| IBIS file generated by  Version 3.24
|   j6plus
[IBIS ver]   5.0
[File name]   j6plus.ibs
[File Rev]   1.0.0
[Date]   Mon Apr 10, 2017, 14:43:27
[Source]   Data created at Texas Instruments
[Notes]   J6Plus 23mm IBIS Model Revision History
   Version 1.0.0, April 10th, 2017
   - Initial Release
   Note 1) Checked by IBISCHK5.
[Disclaimer] Please be aware that in the absence of a written agreement,
   Texas Instruments (TI) assumes no liability for: 1) the
   accuracy of the IBIS models provided to your company, 2) the
   proper functioning of these IBIS models in your design or for
   any resulting applications, or, 3) infringement of patents,
   copyrights, or intellectual property rights resulting from
   your use of these IBIS models. TI provides IBIS models as a
   service to our customers and therefore reserves the right to
   limit distribution of the IBIS models.
[Copyright]   Property of Texas Instruments Incorporated. Unauthorised
   reproduction and/or distribution is strictly prohibited. This
   product is protected under copyright law and trade secret law
   as an unpublished work. Created 2016,(C) Copyright 2016,
   Texas Instruments Incorporated., All Rights Reserved. These
   commodities are under the U.S. Government distribution license
   control.As such,they are not to be re-exported without the
   prior approval of the U.S. Department of Commerce.
|   Component j6plus
[Component]   j6plus
[Manufacturer]   Texas Instruments.
| Source IO level model revisions
|Model   Revision   Date
|DDR_SEIOPB_H   2.5   23 May 2014
|CAMERARX_ADDON   0.9   March 31, 2014
|ACSPCIE_RX   0.5   May 16, 2012
|HDMITXPHY   0.8   Jul 12, 2011
|BC1833DV40DCPBFBP1811_SSCEH   2.0   Sep 11, 2013
|CAMERARX_CORE   0.9   March 31, 2014
|IQ1833DVTCKPBFBP18LL_SSCEV   2.0   Sep 11, 2013
|SDIO1833PB_H   1.0   Sep 21, 2011
|DDR_SEIOPB_V   2.5   23 May 2014
|IHHV1833DVHYP1811_SSCEV   1.0   Dec 24, 2012
|DDR_DIFFIOPB_V   2.5   23 May 2014
|BI2C1833DVFZP18_SSCEV   2.0   Sep 11, 2013
|GANGARX   1   Sep 04, 2012
|SATATX   1.0   Nov 07, 2012
|USB3_PCIEGEN1_PCIEGEN2_TX   1.0   Nov 07, 2012
|DDR_DIFFIOPB_H   2.5   23 May 2014
|BC1833DV40DCPBFBP1811_SSCEV   2.0   Sep 11, 2013
|USB2PHYCORE_HMAV10GS80   0.8   July 13, 2011
|BMLBLVDS18_SSCEH   1.0   Jun 13, 2013
[Package]
|   typ   min   max
R_pkg   0.42369669665272   0.092871   0.97124
L_pkg   2.90117154811716E-009 1.36E-09   4.86E-09
C_pkg   1.52619874476987E-012 8.24E-13   2.21E-12
[Pin]   signal_name   model_name   R_pin   L_pin   C_pin
F6   ATESTV   NC
AC17   CSI2_1_DY2   Selector_15  0.47322   3.10E-09   1.23E-12
AE16   CSI2_0_DY3   Selector_17  0.44019   2.71E-09   1.13E-12
AC13   CSI2_1_DX0   Selector_25  0.46457   2.78E-09   1.07E-12
AF16   CSI2_0_DX1   Selector_13  0.50237   2.99E-09   1.30E-12
AD15   CSI2_1_DX1   Selector_13  0.40521   2.59E-09   1.12E-12
AD17   CSI2_0_DX0   Selector_25  0.3281   2.01E-09   9.66E-13
AF19   CSI2_0_DX2   Selector_13  0.5902   3.45E-09   1.35E-12
AE18   CSI2_0_DY4   Selector_17  0.49636   2.64E-09   1.25E-12
AF17   CSI2_0_DY1   Selector_15  0.50908   3.01E-09   1.32E-12
AD14   CSI2_1_DY1   Selector_15  0.4246   2.63E-09   1.07E-12
AD18   CSI2_0_DY0   Selector_17  0.31895   1.98E-09   9.93E-13
AC16   CSI2_1_DX2   Selector_13  0.47087   3.11E-09   1.25E-12
AE19   CSI2_0_DX4   Selector_25  0.4925   2.76E-09   1.18E-12
AE15   CSI2_0_DX3   Selector_25  0.43712   2.72E-09   1.11E-12
AC14   CSI2_1_DY0   Selector_17  0.46446   2.94E-09   1.04E-12
AF20   CSI2_0_DY2   Selector_15  0.60517   3.60E-09   1.40E-12
E19   DCAN1_TX   Selector_23  0.17732   1.75E-09   1.07E-12
D19   DCAN1_RX   Selector_23  0.29009   2.59E-09   1.21E-12
AA27   DDR1_D20   Selector_24  0.47426   3.29E-09   1.74E-12
AB22   DDR1_VREF0   NC
AA24   DDR1_D21   Selector_24  0.33247   2.23E-09   1.42E-12
AH23   DDR1_CKE   Selector_22  0.54196   3.53E-09   1.79E-12
AC28   DDR1_DQSN1   Selector_26  0.65798   3.81E-09   1.48E-12
V28   DDR1_ECC_D7   Selector_24  0.47152   3.15E-09   1.68E-12
AE24   DDR1_A11   Selector_22  0.35245   2.44E-09   1.42E-12
W25   DDR1_D28   Selector_24  0.28879   2.13E-09   1.29E-12
AF22   DDR1_ODT0   Selector_22  0.40147   2.81E-09   1.44E-12
AB27   DDR1_DQS2   Selector_20  0.67189   3.76E-09   1.46E-12
AE25   DDR1_D13   Selector_24  0.41515   3.01E-09   1.57E-12
Y24   DDR1_D27   Selector_24  0.30467   2.05E-09   1.31E-12
AC27   DDR1_DQS1   Selector_20  0.67176   3.88E-09   1.45E-12
V25   DDR1_ECC_D2   Selector_24  0.35131   2.67E-09   1.44E-12
AF23   DDR1_RST   Selector_22  0.45466   3.02E-09   1.62E-12
AG23   DDR1_A8   Selector_22  0.42684   3.00E-09   1.61E-12
AB24   DDR1_D8   Selector_24  0.35689   2.67E-09   1.36E-12
AG26   DDR1_DQM0   Selector_11  0.64729   3.91E-09   2.00E-12
T27   DDR1_DQM_ECC   Selector_11  0.43684   3.03E-09   1.55E-12
AD28   DDR1_D11   Selector_24  0.53861   3.60E-09   1.82E-12
AE22   DDR1_A0   Selector_22  0.35492   2.49E-09   1.43E-12
AH25   DDR1_DQS0   Selector_20  0.68056   3.82E-09   1.46E-12
AC24   DDR1_DQM1   Selector_11  0.35873   2.52E-09   1.41E-12
AF21   DDR1_A13   Selector_22  0.38573   2.77E-09   1.62E-12
AG20   DDR1_A15   Selector_22  0.4557   3.04E-09   1.63E-12
AE20   DDR1_BA0   Selector_22  0.29234   2.04E-09   1.32E-12
AA28   DDR1_D19   Selector_24  0.49032   3.42E-09   1.85E-12
Y27   DDR1_DQM3   Selector_11  0.46763   3.07E-09   1.69E-12
AG21   DDR1_A12   Selector_22  0.38719   2.86E-09   1.64E-12
AG19   DDR1_CASN   Selector_22  0.42733   2.78E-09   1.62E-12
AD20   DDR1_A1   Selector_22  0.21926   1.63E-09   1.17E-12
AB25   DDR1_D17   Selector_24  0.40252   2.71E-09   1.56E-12
T28   DDR1_ECC_D5   Selector_24  0.44485   3.30E-09   1.71E-12
V26   DDR1_ECC_D3   Selector_24  0.33355   2.36E-09   1.48E-12
V24   DDR1_D26   Selector_24  0.26466   2.00E-09   1.29E-12
AF25   DDR1_D4   Selector_24  0.45643   3.11E-09   1.58E-12
AB26   DDR1_DQM2   Selector_11  0.41898   2.75E-09   1.59E-12
AD24   DDR1_A6   Selector_22  0.35013   2.68E-09   1.63E-12
AG22   DDR1_WEN   Selector_22  0.42447   2.86E-09   1.58E-12
AE27   DDR1_D1   Selector_24  0.52049   3.42E-09   1.76E-12
AC26   DDR1_D15   Selector_24  0.41191   2.78E-09   1.58E-12
T26   DDR1_ECC_D6   Selector_24  0.34602   2.50E-09   1.43E-12
AD25   DDR1_D14   Selector_24  0.39609   2.83E-09   1.50E-12
AE21   DDR1_A2   Selector_22  0.28785   2.13E-09   1.21E-12
AC22   DDR1_A7   Selector_22  0.22439   1.72E-09   1.21E-12
AF26   DDR1_D7   Selector_24  0.45878   3.16E-09   1.64E-12
AF28   DDR1_D2   Selector_24  0.62581   3.95E-09   1.94E-12
AB23   DDR1_D25   Selector_24  0.34495   2.49E-09   1.54E-12
U26   DDR1_ECC_D1   Selector_24  0.34279   2.39E-09   1.49E-12
AH24   DDR1_NCK   Selector_1   0.6371   3.54E-09   1.68E-12
U27   DDR1_DQS_ECC   Selector_20  0.5902   3.35E-09   1.36E-12
AE26   DDR1_D0   Selector_24  0.50411   3.40E-09   1.67E-12
AD23   DDR1_CSN0   Selector_22  0.31244   2.34E-09   1.50E-12
AD22   DDR1_A3   Selector_22  0.27077   2.08E-09   1.24E-12
W24   DDR1_D30   Selector_24  0.3292   2.27E-09   1.37E-12
AC25   DDR1_D22   Selector_24  0.46439   3.12E-09   1.76E-12
AH22   DDR1_A5   Selector_22  0.48585   3.28E-09   1.74E-12
AG24   DDR1_CK   Selector_6   0.63186   3.52E-09   1.69E-12
AB28   DDR1_DQSN2   Selector_26  0.66433   3.80E-09   1.48E-12
AD26   DDR1_D12   Selector_24  0.44133   3.15E-09   1.59E-12
AF27   DDR1_D6   Selector_24  0.53391   3.62E-09   1.76E-12
V27   DDR1_ECC_D4   Selector_24  0.41597   2.89E-09   1.57E-12
AE23   DDR1_A4   Selector_22  0.37808   2.74E-09   1.49E-12
U25   DDR1_ECC_D0   Selector_24  0.30068   2.13E-09   1.30E-12
AF24   DDR1_A9   Selector_22  0.39658   2.69E-09   1.50E-12
AH26   DDR1_D3   Selector_24  0.58696   3.71E-09   1.90E-12
AE28   DDR1_D10   Selector_24  0.59778   3.95E-09   1.91E-12
W26   DDR1_D24   Selector_24  0.41375   2.90E-09   1.50E-12
Y28   DDR1_D31   Selector_24  0.48908   3.29E-09   1.77E-12
AD21   DDR1_A10   Selector_22  0.18857   1.54E-09   1.06E-12
AH20   DDR1_RASN   Selector_22  0.45523   2.97E-09   1.68E-12
AG27   DDR1_D5   Selector_24  0.5732   3.45E-09   1.89E-12
AA25   DDR1_D16   Selector_24  0.40361   2.85E-09   1.49E-12
AC23   DDR1_A14   Selector_22  0.36157   2.89E-09   1.65E-12
AH21   DDR1_BA2   Selector_22  0.50674   3.32E-09   1.77E-12
Y26   DDR1_D23   Selector_24  0.30563   2.40E-09   1.43E-12
AG25   DDR1_DQSN0   Selector_26  0.66118   3.82E-09   1.45E-12
Y25   DDR1_D29   Selector_24  0.33786   2.36E-09   1.34E-12
AA26   DDR1_D18   Selector_24  0.40984   2.78E-09   1.59E-12
U28   DDR1_DQSN_ECC   Selector_26  0.58142   3.43E-09   1.36E-12
AD27   DDR1_D9   Selector_24  0.46233   3.31E-09   1.75E-12
W27   DDR1_DQSN3   Selector_26  0.62804   3.57E-09   1.42E-12
W28   DDR1_DQS3   Selector_20  0.65151   3.67E-09   1.43E-12
AC21   DDR1_BA1   Selector_22  0.20841   1.95E-09   1.21E-12
P23   DDR2_A5   Selector_11  0.19884   1.81E-09   1.27E-12
M24   DDR2_BA2   Selector_11  0.38561   3.08E-09   1.66E-12
H25   DDR2_D21   Selector_24  0.32873   2.40E-09   1.46E-12
B27   DDR2_D5   Selector_24  0.52339   3.75E-09   2.03E-12
H27   DDR2_D22   Selector_24  0.44149   3.11E-09   1.66E-12
N24   DDR2_A14   Selector_11  0.20496   1.86E-09   1.20E-12
T25   DDR2_CASN   Selector_11  0.2726   2.24E-09   1.19E-12
R24   DDR2_A13   Selector_11  0.19051   1.48E-09   1.02E-12
R25   DDR2_CKE   Selector_11  0.32341   2.57E-09   1.33E-12
J28   DDR2_DQSN2   Selector_26  0.59604   3.55E-09   1.37E-12
E25   DDR2_D9   Selector_24  0.36266   2.71E-09   1.47E-12
R28   DDR2_CK   Selector_14  0.63061   3.59E-09   1.61E-12
K24   DDR2_D30   Selector_24  0.22548   2.13E-09   1.35E-12
G27   DDR2_D11   Selector_24  0.43022   3.03E-09   1.58E-12
K26   DDR2_D25   Selector_24  0.36091   2.55E-09   1.44E-12
L28   DDR2_DQS3   Selector_20  0.62529   3.80E-09   1.40E-12
J24   DDR2_D29   Selector_24  0.27245   2.16E-09   1.35E-12
N25   DDR2_RST   Selector_11  0.33044   2.79E-09   1.43E-12
J25   DDR2_D26   Selector_24  0.35274   2.47E-09   1.39E-12
T24   DDR2_WEN   Selector_11  0.23939   1.92E-09   1.18E-12
J27   DDR2_DQS2   Selector_20  0.604   3.52E-09   1.34E-12
P26   DDR2_A1   Selector_11  0.35121   2.52E-09   1.45E-12
H24   DDR2_D28   Selector_24  0.33905   2.66E-09   1.59E-12
N26   DDR2_A6   Selector_11  0.3636   2.64E-09   1.45E-12
F27   DDR2_DQS1   Selector_20  0.7305   4.09E-09   1.57E-12
L25   DDR2_A10   Selector_11  0.3358   2.53E-09   1.53E-12
D26   DDR2_D4   Selector_24  0.44637   3.26E-09   1.60E-12
R26   DDR2_RASN   Selector_11  0.32251   2.49E-09   1.34E-12
K28   DDR2_D27   Selector_24  0.47179   3.20E-09   1.69E-12
R23   DDR2_A15   Selector_11  0.17102   1.42E-09   9.48E-13
M27   DDR2_A9   Selector_11  0.4387   3.07E-09   1.64E-12
D25   DDR2_D3   Selector_24  0.39925   2.89E-09   1.49E-12
K27   DDR2_D24   Selector_24  0.45334   3.19E-09   1.58E-12
D27   DDR2_DQSN0   Selector_26  0.68594   3.95E-09   1.46E-12
P28   DDR2_A2   Selector_11  0.4806   3.52E-09   1.80E-12
J26   DDR2_DQM3   Selector_11  0.42358   3.15E-09   1.66E-12
H28   DDR2_D20   Selector_24  0.49628   3.66E-09   1.84E-12
P27   DDR2_A3   Selector_11  0.40859   2.90E-09   1.58E-12
G24   DDR2_D17   Selector_24  0.35079   2.66E-09   1.60E-12
P25   DDR2_A0   Selector_11  0.26462   2.02E-09   1.23E-12
A26   DDR2_D1   Selector_24  0.50901   3.87E-09   2.00E-12
E24   DDR2_D2   Selector_24  0.38689   2.96E-09   1.52E-12
U24   DDR2_BA1   Selector_11  0.26815   2.12E-09   1.21E-12
C26   DDR2_D7   Selector_24  0.45744   3.30E-09   1.76E-12
M22   DDR2_VREF0   NC
M25   DDR2_A7   Selector_11  0.26291   2.06E-09   1.30E-12
F24   DDR2_D19   Selector_24  0.34822   2.79E-09   1.70E-12
G23   DDR2_DQM2   Selector_11  0.27859   2.26E-09   1.57E-12
C28   DDR2_D0   Selector_24  0.62669   4.38E-09   2.04E-12
M26   DDR2_CSN0   Selector_11  0.33733   2.53E-09   1.55E-12
F26   DDR2_D8   Selector_24  0.43184   3.11E-09   1.46E-12
P24   DDR2_A4   Selector_11  0.20852   1.74E-09   1.08E-12
E26   DDR2_D10   Selector_24  0.45673   3.22E-09   1.56E-12
F23   DDR2_D18   Selector_24  0.32703   2.83E-09   1.75E-12
B26   DDR2_D6   Selector_24  0.50709   3.63E-09   1.97E-12
E28   DDR2_D12   Selector_24  0.57819   3.92E-09   1.81E-12
D28   DDR2_DQS0   Selector_20  0.71828   4.02E-09   1.50E-12
N28   DDR2_A8   Selector_11  0.48119   3.33E-09   1.70E-12
K25   DDR2_ODT0   Selector_11  0.445   3.37E-09   1.86E-12
L27   DDR2_DQSN3   Selector_26  0.60186   3.60E-09   1.43E-12
G25   DDR2_D16   Selector_24  0.41288   3.08E-09   1.71E-12
F28   DDR2_DQSN1   Selector_26  0.73785   4.21E-09   1.57E-12
G28   DDR2_D14   Selector_24  0.4674   3.37E-09   1.76E-12
L26   DDR2_D31   Selector_24  0.34691   2.45E-09   1.41E-12
N27   DDR2_A11   Selector_11  0.38845   2.75E-09   1.51E-12
H26   DDR2_D23   Selector_24  0.37415   2.64E-09   1.56E-12
F25   DDR2_D15   Selector_24  0.34955   2.65E-09   1.39E-12
C27   DDR2_DQM0   Selector_11  0.5469   4.01E-09   1.82E-12
L24   DDR2_BA0   Selector_11  0.2659   2.36E-09   1.44E-12
G26   DDR2_D13   Selector_24  0.38989   2.74E-09   1.55E-12
E27   DDR2_DQM1   Selector_11  0.55797   3.78E-09   1.97E-12
M28   DDR2_A12   Selector_11  0.47329   3.27E-09   1.73E-12
R27   DDR2_NCK   Selector_27  0.61545   3.53E-09   1.63E-12
F19   EMU0   Selector_23  0.13176   1.42E-09   8.78E-13
C23   EMU1   Selector_23  0.51333   3.38E-09   1.80E-12
F17   GPIO6_15   Selector_23  0.19784   1.98E-09   1.08E-12
AB4   GPIO6_11   Selector_4   0.46323   2.99E-09   1.77E-12
AC5   GPIO6_10   Selector_4   0.61618   3.82E-09   2.06E-12
F18   GPIO6_16   Selector_23  0.15426   1.52E-09   9.50E-13
E21   GPIO6_14   Selector_23  0.25374   2.28E-09   1.07E-12
R1   GPMC_A18   Selector_4   0.49354   3.50E-09   1.72E-12
M5   GPMC_OEN_REN   Selector_4   0.25199   2.05E-09   1.12E-12
H5   GPMC_A27   Selector_4   0.22331   1.86E-09   1.13E-12
P6   GPMC_A0   Selector_4   0.18008   1.52E-09   1.09E-12
L5   GPMC_AD2   Selector_4   0.26493   2.15E-09   1.15E-12
M4   GPMC_BEN1   Selector_4   0.28629   2.30E-09   1.24E-12
K2   GPMC_AD13   Selector_4   0.36396   2.68E-09   1.47E-12
T2   GPMC_A15   Selector_4   0.53356   3.66E-09   1.78E-12
L1   GPMC_AD8   Selector_4   0.50617   3.58E-09   1.67E-12
H4   GPMC_A25   Selector_4   0.28037   2.27E-09   1.33E-12
J2   GPMC_AD11   Selector_4   0.42103   3.01E-09   1.57E-12
K6   GPMC_AD4   Selector_4   0.23005   1.89E-09   1.10E-12
M2   GPMC_AD1   Selector_4   0.41338   3.06E-09   1.55E-12
J1   GPMC_AD10   Selector_4   0.498   3.50E-09   1.70E-12
P3   GPMC_A17   Selector_4   0.41172   2.97E-09   1.54E-12
G4   GPMC_CS1   Selector_4   0.26966   2.20E-09   1.26E-12
M1   GPMC_AD3   Selector_4   0.48001   3.52E-09   1.67E-12
G5   GPMC_A23   Selector_4   0.22275   2.08E-09   1.21E-12
R4   GPMC_A2   Selector_4   0.34771   2.60E-09   1.14E-12
J5   GPMC_A10   Selector_4   0.22191   2.40E-09   1.28E-12
M3   GPMC_WEN   Selector_4   0.34292   2.82E-09   1.36E-12
H1   GPMC_AD12   Selector_4   0.5391   3.75E-09   1.75E-12
N4   GPMC_A8   Selector_4   0.27934   2.32E-09   1.23E-12
L4   GPMC_AD5   Selector_4   0.25799   2.02E-09   1.23E-12
N2   GPMC_WAIT0   Selector_4   0.41982   3.14E-09   1.53E-12
N5   GPMC_AD0   Selector_4   0.40226   3.08E-09   1.52E-12
J6   GPMC_A1   Selector_4   0.23468   2.46E-09   1.24E-12
H6   GPMC_A19   Selector_4   0.15553   1.39E-09   8.82E-13
H2   GPMC_AD14   Selector_4   0.49023   3.33E-09   1.65E-12
P2   GPMC_CS2   Selector_4   0.43903   3.14E-09   1.57E-12
U1   GPMC_A16   Selector_4   0.54425   3.76E-09   1.82E-12
H3   GPMC_A26   Selector_4   0.31252   2.45E-09   1.40E-12
J3   GPMC_A24   Selector_4   0.31402   2.52E-09   1.35E-12
F5   GPMC_A22   Selector_4   0.28715   2.79E-09   1.47E-12
K5   GPMC_A11   Selector_4   0.23539   2.44E-09   1.27E-12
N6   GPMC_A7   Selector_4   0.17847   1.50E-09   1.02E-12
R2   GPMC_A13   Selector_4   0.43208   3.16E-09   1.59E-12
L2   GPMC_AD7   Selector_4   0.40505   2.94E-09   1.55E-12
K3   GPMC_AD15   Selector_4   0.30569   2.36E-09   1.34E-12
G6   GPMC_A20   Selector_4   0.22002   1.98E-09   1.24E-12
R3   GPMC_A9   Selector_4   0.40041   2.92E-09   1.50E-12
K4   GPMC_A5   Selector_4   0.31091   2.86E-09   1.40E-12
J4   GPMC_A21   Selector_4   0.24739   2.01E-09   1.27E-12
L3   GPMC_AD6   Selector_4   0.38163   2.77E-09   1.43E-12
N3   GPMC_BEN0   Selector_4   0.29182   2.53E-09   1.32E-12
K1   GPMC_AD9   Selector_4   0.40967   2.97E-09   1.58E-12
R5   GPMC_A3   Selector_4   0.26198   2.01E-09   1.09E-12
P1   GPMC_CS3   Selector_4   0.54568   3.87E-09   1.77E-12
P5   GPMC_A6   Selector_4   0.34047   2.61E-09   1.32E-12
R6   GPMC_A14   Selector_4   0.44443   3.33E-09   1.69E-12
P4   GPMC_A12   Selector_4   0.29397   2.27E-09   1.32E-12
L6   GPMC_CLK   Selector_4   0.16087   1.50E-09   1.26E-12
M6   GPMC_A4   Selector_4   0.15466   1.38E-09   1.02E-12
N1   GPMC_ADVN_ALE   Selector_4   0.52762   3.88E-09   1.73E-12
T1   GPMC_CS0   Selector_4   0.5994   4.10E-09   1.89E-12
AG14   HDMI1_CLOCKX   ibis_tmdsp_M#336   0.55573   2.99E-09   1.37E-12
AH18   HDMI1_DATA1Y   ibis_tmdsm_M#337   0.59298   3.19E-09   1.39E-12
AG18   HDMI1_DATA2X   ibis_tmdsp_M#336   0.56768   3.10E-09   1.28E-12
AH16   HDMI1_DATA0Y   ibis_tmdsm_M#337   0.52675   2.88E-09   1.32E-12
AG15   HDMI1_DATA0X   ibis_tmdsp_M#336   0.52784   2.86E-09   1.33E-12
AG17   HDMI1_DATA1X   ibis_tmdsp_M#336   0.56542   3.06E-09   1.37E-12
AH19   HDMI1_DATA2Y   ibis_tmdsm_M#337   0.58397   3.26E-09   1.31E-12
AH15   HDMI1_CLOCKY   ibis_tmdsm_M#337   0.55862   3.05E-09   1.37E-12
C19   I2C1_SCL   Selector_16  0.37854   2.73E-09   1.57E-12
C20   I2C1_SDA   Selector_16  0.41108   2.82E-09   1.55E-12
F15   I2C2_SCL   Selector_16  0.24519   2.03E-09   1.36E-12
C24   I2C2_SDA   Selector_16  0.56681   3.51E-09   1.90E-12
B28   IFORCE   NC
AF14   LJCB_CLKN   ACSPCIE_RX_M#335   0.3515   1.98E-09   1.29E-12
AE13   LJCB_CLKP   ACSPCIE_RX_M#335   0.35246   1.95E-09   1.29E-12
C12   MCASP1_AXR10   Selector_23  0.33446   2.49E-09   1.47E-12
D14   MCASP1_AXR12   Selector_23  0.22318   1.95E-09   1.22E-12
E12   MCASP1_AXR4   Selector_23  0.21323   1.78E-09   1.17E-12
D13   MCASP1_AXR5   Selector_23  0.23567   2.08E-09   1.21E-12
B12   MCASP1_AXR13   Selector_23  0.42421   3.04E-09   1.58E-12
B11   MCASP1_AXR8   Selector_23  0.38326   2.96E-09   1.57E-12
E14   MCASP1_AXR15   Selector_23  0.24085   1.99E-09   1.16E-12
A12   MCASP1_AXR11   Selector_23  0.45509   3.30E-09   1.65E-12
A11   MCASP1_AXR9   Selector_23  0.46183   3.35E-09   1.68E-12
E11   MCASP1_AXR3   Selector_23  0.25365   2.05E-09   1.24E-12
D12   MCASP1_AXR7   Selector_23  0.30704   2.35E-09   1.28E-12
B13   MCASP1_ACLKX   Selector_23  0.38146   2.87E-09   1.53E-12
C11   MCASP1_AXR6   Selector_23  0.32814   2.57E-09   1.43E-12
F11   MCASP1_AXR1   Selector_23  0.21935   1.87E-09   1.14E-12
C13   MCASP1_FSX   Selector_23  0.26929   2.19E-09   1.39E-12
F14   MCASP1_FSR   Selector_23  0.18526   1.56E-09   1.07E-12
A13   MCASP1_ACLKR   Selector_23  0.42105   3.00E-09   1.63E-12
E13   MCASP1_AXR2   Selector_23  0.092871   1.38E-09   8.93E-13
F12   MCASP1_AXR14   Selector_23  0.17677   1.62E-09   8.24E-13
F10   MCASP1_AXR0   Selector_23  0.18905   1.82E-09   1.19E-12
A17   MCASP2_FSX   Selector_23  0.58524   3.96E-09   2.02E-12
A19   MCASP2_FSR   Selector_23  0.65208   4.23E-09   2.18E-12
A16   MCASP2_AXR7   Selector_23  0.552   3.72E-09   1.93E-12
B14   MCASP2_AXR0   Selector_23  0.39699   2.82E-09   1.66E-12
B15   MCASP2_AXR5   Selector_23  0.44426   3.16E-09   1.66E-12
A14   MCASP2_AXR1   Selector_23  0.50121   3.46E-09   1.75E-12
D15   MCASP2_AXR4   Selector_23  0.28214   2.20E-09   1.35E-12
A15   MCASP2_AXR3   Selector_23  0.48973   3.34E-09   1.74E-12
C14   MCASP2_AXR2   Selector_23  0.32212   2.37E-09   1.39E-12
A18   MCASP2_ACLKX   Selector_23  0.53013   3.51E-09   1.84E-12
B16   MCASP2_AXR6   Selector_23  0.39   2.84E-09   1.58E-12
E15   MCASP2_ACLKR   Selector_23  0.1899   1.46E-09   1.15E-12
B18   MCASP3_AXR0   Selector_23  0.41165   2.85E-09   1.57E-12
B17   MCASP3_ACLKX   Selector_23  0.42894   2.91E-09   1.63E-12
C16   MCASP3_AXR1   Selector_23  0.34144   2.49E-09   1.45E-12
F13   MCASP3_FSX   Selector_23  0.23996   2.05E-09   1.21E-12
A20   MCASP4_FSX   Selector_23  0.52153   3.48E-09   1.82E-12
D17   MCASP4_AXR1   Selector_23  0.27464   2.06E-09   1.30E-12
D16   MCASP4_AXR0   Selector_23  0.16794   1.84E-09   1.18E-12
C17   MCASP4_ACLKX   Selector_23  0.4215   2.91E-09   1.52E-12
AB6   MCASP5_FSX   Selector_4   0.41465   2.73E-09   1.58E-12
AA4   MCASP5_AXR1   Selector_4   0.43954   2.86E-09   1.74E-12
AB3   MCASP5_AXR0   Selector_4   0.46779   3.05E-09   1.77E-12
AA3   MCASP5_ACLKX   Selector_4   0.4844   3.22E-09   1.67E-12
V1   MDIO_MCLK   Selector_4   0.57447   3.80E-09   1.90E-12
U3   MDIO_D   Selector_4   0.38305   2.58E-09   1.53E-12
AB1   MLBP_CLK_P   Selector_2   0.7668   4.20E-09   1.85E-12
AA2   MLBP_DAT_N   Selector_9   0.72941   4.04E-09   1.52E-12
AB2   MLBP_CLK_N   Selector_2   0.76043   4.14E-09   1.83E-12
AC2   MLBP_SIG_N   Selector_9   0.78823   4.31E-09   1.59E-12
AA1   MLBP_DAT_P   Selector_9   0.72772   4.13E-09   1.51E-12
AC1   MLBP_SIG_P   Selector_9   0.80114   4.31E-09   1.63E-12
V6   MMC1_SDWP   Selector_4   0.19952   1.46E-09   1.16E-12
W3   MMC1_CLK   Selector_5   0.36035   2.56E-09   1.58E-12
W4   MMC1_SDCD   Selector_4   0.31882   2.24E-09   1.44E-12
Y4   MMC1_DAT1   Selector_5   0.40029   2.71E-09   1.67E-12
V5   MMC1_DAT0   Selector_5   0.31001   2.32E-09   1.34E-12
Y3   MMC1_DAT3   Selector_5   0.42805   2.91E-09   1.61E-12
W5   MMC1_CMD   Selector_5   0.31704   2.16E-09   1.41E-12
Y5   MMC1_DAT2   Selector_5   0.39546   2.74E-09   1.64E-12
AB7   MMC3_DAT6   Selector_4   0.43055   2.92E-09   1.71E-12
AC6   MMC3_DAT2   Selector_4   0.46203   3.07E-09   1.66E-12
AC7   MMC3_CMD   Selector_4   0.5286   3.64E-09   1.84E-12
AC4   MMC3_DAT3   Selector_4   0.57319   3.45E-09   1.95E-12
AA5   MMC3_DAT7   Selector_4   0.35903   2.41E-09   1.52E-12
AA6   MMC3_DAT4   Selector_4   0.37993   2.63E-09   1.52E-12
AC3   MMC3_CLK   Selector_4   0.49296   3.15E-09   1.75E-12
AB5   MMC3_DAT5   Selector_4   0.38564   2.57E-09   1.54E-12
Y6   MMC3_DAT0   Selector_4   0.25419   1.80E-09   1.28E-12
W6   MMC3_DAT1   Selector_4   0.20733   1.58E-09   1.17E-12
AH9   PCIE_RXP1   usb3rx_M#715   0.65527   3.53E-09   1.47E-12
AG9   PCIE_TXN1   Selector_7   0.59952   3.27E-09   1.45E-12
AG12   PCIE_TXN0   Selector_7   0.52323   2.85E-09   1.33E-12
AH10   PCIE_TXP1   Selector_21  0.60849   3.34E-09   1.42E-12
AG11   PCIE_RXN0   usb3rx_M#715   0.52095   2.80E-09   1.33E-12
AG8   PCIE_RXN1   usb3rx_M#715   0.64833   3.44E-09   1.48E-12
AH12   PCIE_RXP0   usb3rx_M#715   0.52941   2.89E-09   1.33E-12
AH13   PCIE_TXP0   Selector_21  0.53798   2.89E-09   1.34E-12
C25   PORZ   Selector_18  0.53951   3.88E-09   1.78E-12
D24   RESETN   Selector_8   0.51082   3.80E-09   1.67E-12
T5   RGMII0_TXD0   Selector_4   0.2657   2.11E-09   1.25E-12
U4   RGMII0_RXC   Selector_4   0.40317   2.79E-09   1.56E-12
Y2   RGMII0_RXD1   Selector_4   0.59491   3.80E-09   1.90E-12
V4   RGMII0_RXCTL   Selector_4   0.40168   2.84E-09   1.60E-12
T4   RGMII0_TXD3   Selector_4   0.27961   2.19E-09   1.37E-12
W2   RGMII0_RXD3   Selector_4   0.5259   3.73E-09   1.81E-12
W1   RGMII0_RXD0   Selector_4   0.53313   3.74E-09   1.92E-12
T3   RGMII0_TXD2   Selector_4   0.34803   2.80E-09   1.51E-12
T6   RGMII0_TXC   Selector_4   0.18507   1.46E-09   1.13E-12
U5   RGMII0_TXCTL   Selector_4   0.33553   2.42E-09   1.33E-12
U6   RGMII0_TXD1   Selector_4   0.37411   2.67E-09   1.57E-12
V3   RGMII0_RXD2   Selector_4   0.44923   3.04E-09   1.70E-12
U2   RMII_MHZ_50_CLK   Selector_4   0.49781   3.29E-09   1.77E-12
D23   RSTOUTN   Selector_3   0.47264   3.40E-09   1.74E-12
E18   RTCK   Selector_3   0.20614   1.61E-09   1.14E-12
AG6   SATA1_TXN0   sata_tx_M#759   0.73959   3.93E-09   1.62E-12
AG5   SATA1_RXP0   usb3rx_M#715   0.83495   4.37E-09   1.75E-12
AH6   SATA1_RXN0   usb3rx_M#715   0.82304   4.33E-09   1.76E-12
AH7   SATA1_TXP0   sata_tx_M#759   0.7495   3.93E-09   1.61E-12
C15   SPI1_D1   Selector_23  0.17598   2.47E-09   1.35E-12
A21   SPI1_CS1   Selector_23  0.59228   3.79E-09   2.03E-12
B19   SPI1_CS3   Selector_23  0.47701   3.52E-09   1.86E-12
B24   SPI1_D0   Selector_23  0.34305   4.18E-09   2.17E-12
B20   SPI1_CS2   Selector_23  0.48542   3.52E-09   1.79E-12
A23   SPI1_CS0   Selector_23  0.62624   4.18E-09   2.08E-12
A24   SPI1_SCLK   Selector_23  0.70609   4.38E-09   2.17E-12
B23   SPI2_CS0   Selector_23  0.62835   3.92E-09   2.04E-12
E16   SPI2_D0   Selector_23  0.1358   1.46E-09   1.14E-12
B21   SPI2_D1   Selector_23  0.54119   3.70E-09   1.85E-12
A25   SPI2_SCLK   Selector_23  0.73945   4.49E-09   2.21E-12
E20   TCLK   Selector_12  0.23692   2.02E-09   1.14E-12
B22   TDI   Selector_8   0.44949   3.00E-09   1.76E-12
C18   TDO   Selector_3   0.27882   2.66E-09   1.29E-12
F16   TMS   Selector_23  0.20144   1.88E-09   1.16E-12
D20   TRSTN   Selector_8   0.30933   2.49E-09   1.30E-12
F22   UART1_RXD   Selector_23  0.24211   2.17E-09   1.16E-12
C21   UART1_TXD   Selector_23  0.32924   2.79E-09   1.40E-12
E23   UART1_RTSN   Selector_23  0.34686   2.62E-09   1.37E-12
F21   UART1_CTSN   Selector_23  0.20632   1.66E-09   1.07E-12
E22   UART2_TXD   Selector_23  0.23784   1.94E-09   1.14E-12
F20   UART2_CTSN   Selector_23  0.20323   1.86E-09   1.09E-12
C22   UART2_RTSN   Selector_23  0.32321   2.75E-09   1.38E-12
D22   UART2_RXD   Selector_23  0.29936   2.49E-09   1.32E-12
Y1   UART3_TXD   Selector_4   0.60251   3.97E-09   1.99E-12
V2   UART3_RXD   Selector_4   0.50843   3.55E-09   1.81E-12
AG3   USB_RXN0   usb3rx_M#715   0.88739   4.58E-09   1.87E-12
AH4   USB_RXP0   usb3rx_M#715   0.90023   4.58E-09   1.88E-12
AH3   USB_TXP0   Selector_21  0.97124   4.86E-09   1.94E-12
AG2   USB_TXN0   Selector_7   0.96382   4.81E-09   1.93E-12
AF11   USB1_DP   Selector_10  0.34196   2.14E-09   1.16E-12
AD12   USB1_DRVVBUS   Selector_4   0.27037   2.08E-09   1.49E-12
AE10   USB1_DM   Selector_19  0.3484   2.16E-09   1.09E-12
AC11   USB2_DRVVBUS   Selector_4   0.20922   1.59E-09   1.29E-12
AF13   USB2_DM   Selector_19  0.33442   2.44E-09   1.41E-12
AE12   USB2_DP   Selector_10  0.34279   2.52E-09   1.42E-12
AF8   VIN1A_D6   Selector_4   0.47218   3.01E-09   1.71E-12
AE6   VIN1A_D4   Selector_4   0.38178   2.46E-09   1.57E-12
AE2   VIN1A_D21   Selector_4   0.60479   3.71E-09   1.97E-12
AE4   VIN1A_D16   Selector_4   0.49785   3.17E-09   1.77E-12
AE9   VIN1A_D0   Selector_4   0.42578   2.83E-09   1.61E-12
AF4   VIN1A_D8   Selector_4   0.51129   3.11E-09   1.84E-12
AD5   VIN1A_D18   Selector_4   0.40175   2.64E-09   1.59E-12
AE5   VIN1A_D12   Selector_4   0.43868   2.82E-09   1.69E-12
AD9   VIN1A_FLD0   Selector_4   0.3729   2.41E-09   1.48E-12
AE7   VIN1A_D2   Selector_4   0.34628   2.31E-09   1.46E-12
AF5   VIN1A_D11   Selector_4   0.50781   3.21E-09   1.78E-12
AD8   VIN1A_CLK0   Selector_4   0.28716   2.02E-09   1.28E-12
AD4   VIN1A_D20   Selector_4   0.47523   3.21E-09   1.66E-12
AE3   VIN1A_D15   Selector_4   0.529   3.31E-09   1.85E-12
AE1   VIN1A_D17   Selector_4   0.63023   3.89E-09   2.04E-12
AF10   VIN1A_D1   Selector_4   0.43066   2.73E-09   1.83E-12
AF3   VIN1A_D10   Selector_4   0.58198   3.57E-09   1.92E-12
AF7   VIN1A_D5   Selector_4   0.43511   2.66E-09   1.68E-12
AF6   VIN1A_D7   Selector_4   0.46497   2.87E-09   1.71E-12
AC9   VIN1A_DE0   Selector_4   0.24694   1.65E-09   1.25E-12
AD7   VIN1A_VSYNC0   Selector_4   0.28751   1.98E-09   1.35E-12
AF1   VIN1A_D13   Selector_4   0.71399   4.30E-09   2.18E-12
AD3   VIN1A_D19   Selector_4   0.50355   3.31E-09   1.77E-12
AD6   VIN1A_D14   Selector_4   0.41802   2.84E-09   1.57E-12
AC8   VIN1B_CLK1   Selector_4   0.17211   1.36E-09   1.11E-12
AD2   VIN1A_D23   Selector_4   0.57315   3.77E-09   1.90E-12
AD1   VIN1A_D22   Selector_4   0.60708   3.88E-09   1.97E-12
AF2   VIN1A_D9   Selector_4   0.61227   3.68E-09   2.03E-12
AC10   VIN1A_HSYNC0   Selector_4   0.38077   2.48E-09   1.62E-12
AE8   VIN1A_D3   Selector_4   0.39403   2.56E-09   1.54E-12
D5   VIN2A_FLD0   Selector_23  0.21733   2.46E-09   1.33E-12
D4   VIN2A_D18   Selector_23  0.47347   3.15E-09   1.77E-12
C2   VIN2A_D14   Selector_23  0.59052   3.67E-09   1.96E-12
C1   VIN2A_D13   Selector_23  0.58531   3.79E-09   2.02E-12
F2   VIN2A_D0   Selector_23  0.44224   3.14E-09   1.61E-12
E3   VIN2A_D1   Selector_23  0.54156   3.68E-09   1.83E-12
B5   VIN2A_D17   Selector_23  0.45898   3.08E-09   1.75E-12
D1   VIN2A_D6   Selector_23  0.61593   4.02E-09   2.02E-12
C3   VIN2A_D15   Selector_23  0.53585   3.51E-09   1.83E-12
E6   VIN2A_D12   Selector_23  0.4498   3.04E-09   1.66E-12
C5   VIN2A_D9   Selector_23  0.33782   2.68E-09   1.53E-12
E5   VIN2A_VSYNC0   Selector_23  0.2868   2.16E-09   1.30E-12
G3   VIN2A_D8   Selector_23  0.43622   3.33E-09   1.72E-12
F1   VIN2A_CLK0   Selector_23  0.43335   3.22E-09   1.67E-12
E4   VIN2A_D7   Selector_23  0.44717   3.05E-09   1.64E-12
A3   VIN2A_D19   Selector_23  0.65096   3.96E-09   2.06E-12
B3   VIN2A_D20   Selector_23  0.60106   3.77E-09   2.00E-12
D3   VIN2A_D10   Selector_23  0.49103   3.29E-09   1.75E-12
B2   VIN2A_D16   Selector_23  0.64088   3.86E-09   2.06E-12
G2   VIN2A_DE0   Selector_23  0.37363   2.89E-09   1.45E-12
D2   VIN2A_D4   Selector_23  0.49422   3.29E-09   1.82E-12
E2   VIN2A_D3   Selector_23  0.50432   3.38E-09   1.69E-12
F4   VIN2A_D11   Selector_23  0.33172   2.87E-09   1.49E-12
A4   VIN2A_D23   Selector_23  0.5766   3.80E-09   1.95E-12
G1   VIN2A_HSYNC0   Selector_23  0.42591   3.17E-09   1.57E-12
F3   VIN2A_D5   Selector_23  0.44564   3.14E-09   1.72E-12
C4   VIN2A_D22   Selector_23  0.54495   3.62E-09   1.85E-12
B4   VIN2A_D21   Selector_23  0.5983   3.79E-09   1.90E-12
E1   VIN2A_D2   Selector_23  0.61243   3.97E-09   2.00E-12
C9   VOUT1_D20   Selector_23  0.40185   2.79E-09   1.52E-12
A9   VOUT1_D23   Selector_23  0.47345   3.31E-09   1.74E-12
B7   VOUT1_D16   Selector_23  0.541   3.61E-09   1.76E-12
A10   VOUT1_HSYNC   Selector_23  0.47312   3.36E-09   1.72E-12
C10   VOUT1_DE   Selector_23  0.35786   2.65E-09   1.50E-12
A7   VOUT1_D19   Selector_23  0.53525   3.58E-09   1.84E-12
C7   VOUT1_D15   Selector_23  0.4436   3.11E-09   1.59E-12
D6   VOUT1_D10   Selector_23  0.41909   3.24E-09   1.58E-12
F7   VOUT1_D6   Selector_23  0.28336   2.49E-09   1.31E-12
D8   VOUT1_D9   Selector_23  0.34533   2.53E-09   1.45E-12
D10   VOUT1_VSYNC   Selector_23  0.29412   2.34E-09   1.43E-12
F8   VOUT1_D5   Selector_23  0.23364   1.94E-09   1.14E-12
C8   VOUT1_D14   Selector_23  0.40043   2.79E-09   1.58E-12
D11   VOUT1_CLK   Selector_23  0.23889   1.91E-09   1.27E-12
B9   VOUT1_D22   Selector_23  0.43215   2.98E-09   1.65E-12
D7   VOUT1_D11   Selector_23  0.38624   2.85E-09   1.53E-12
B6   VOUT1_D13   Selector_23  0.48769   3.35E-09   1.69E-12
E10   VOUT1_D1   Selector_23  0.16721   1.79E-09   9.90E-13
A6   VOUT1_D18   Selector_23  0.55879   3.75E-09   1.87E-12
A8   VOUT1_D21   Selector_23  0.47576   3.28E-09   1.83E-12
C6   VOUT1_D3   Selector_23  0.41917   3.11E-09   1.51E-12
F9   VOUT1_D0   Selector_23  0.15333   1.41E-09   9.59E-13
D9   VOUT1_D2   Selector_23  0.28356   2.32E-09   1.27E-12
E8   VOUT1_D8   Selector_23  0.2771   2.24E-09   1.25E-12
E7   VOUT1_D7   Selector_23  0.33479   2.54E-09   1.45E-12
B8   VOUT1_D17   Selector_23  0.48946   3.26E-09   1.78E-12
A5   VOUT1_D12   Selector_23  0.58274   3.74E-09   1.91E-12
B10   VOUT1_FLD   Selector_23  0.38792   2.79E-09   1.55E-12
E9   VOUT1_D4   Selector_23  0.23344   1.94E-09   1.12E-12
A27   VSENSE   NC
AB19   WAKEUP0   Selector_18  0.21221   2.31E-09   1.61E-12
AC20   WAKEUP1   Selector_18  0.28021   3.23E-09   1.78E-12
AC19   XI_OSC1   NC
AB16   XI_OSC0   NC
AB14   XO_OSC0   NC
AB18   XO_OSC1   NC
B25   XREF_CLK2   Selector_23  0.6968   4.25E-09   2.10E-12
D18   XREF_CLK0   Selector_23  0.33169   2.32E-09   1.36E-12
E17   XREF_CLK1   Selector_23  0.26843   2.04E-09   1.25E-12
A22   XREF_CLK3   Selector_23  0.59598   3.96E-09   2.00E-12
[Diff Pin] inv_pin vdiff tdelay_typ tdelay_min tdelay_max
|Differential signal data for cell USB2PHYCORE_HMAV10GS80
|USB2_DP   USB2_DM
AE12   AF13   200mV 0ns 0ns 0ns
|USB1_DP   USB1_DM
AF11   AE10   200mV 0ns 0ns 0ns
|Differential signal data for cell BMLBLVDS18_SSCEH
|MLBP_DAT_N   MLBP_DAT_P
AA2   AA1   200m   NA
|MLBP_CLK_P   MLBP_CLK_N
AB1   AB2   200m   NA
|MLBP_SIG_P   MLBP_SIG_N
AC1   AC2   200m   NA
|Differential signal data for cell DDR_DIFFIOPB_V
|DDR1_CK   DDR1_NCK
AG24   AH24   200m   0
|Differential signal data for cell DDR_DIFFIOPB_H
|DDR1_DQS_ECC   DDR1_DQSN_ECC
U27   U28   200m   0
|DDR1_DQS2   DDR1_DQSN2
AB27   AB28   200m   0
|DDR2_DQS3   DDR2_DQSN3
L28   L27   200m   0
|DDR1_DQS1   DDR1_DQSN1
AC27   AC28   200m   0
|DDR1_DQS3   DDR1_DQSN3
W28   W27   200m   0
|DDR1_DQS0   DDR1_DQSN0
AH25   AG25   200m   0
|DDR2_DQS0   DDR2_DQSN0
D28   D27   200m   0
|DDR2_DQS2   DDR2_DQSN2
J27   J28   200m   0
|DDR2_DQS1   DDR2_DQSN1
F27   F28   200m   0
|DDR2_CK   DDR2_NCK
R28   R27   200m   0
|Differential signal data for cell CAMERARX_CORE
|CSI2_1_DX1   CSI2_1_DY1
AD15   AD14   200m   NA
|CSI2_0_DX2   CSI2_0_DY2
AF19   AF20   200m   NA
|CSI2_1_DX2   CSI2_1_DY2
AC16   AC17   200m   NA
|CSI2_0_DX1   CSI2_0_DY1
AF16   AF17   200m   NA
|Differential signal data for cell SATATX
|SATA1_TXP0   SATA1_TXN0
AH7   AG6   200m   0
|Differential signal data for cell USB3_PCIEGEN1_PCIEGEN2_TX
|PCIE_TXP0   PCIE_TXN0
AH13   AG12   200m   0
|PCIE_TXP1   PCIE_TXN1
AH10   AG9   200m   0
|USB_TXP0   USB_TXN0
AH3   AG2   200m   0
|Differential signal data for cell CAMERARX_ADDON
|CSI2_0_DX0   CSI2_0_DY0
AD17   AD18   200m   NA
|CSI2_0_DX4   CSI2_0_DY4
AE19   AE18   200m   NA
|CSI2_0_DX3   CSI2_0_DY3
AE15   AE16   200m   NA
|CSI2_1_DX0   CSI2_1_DY0
AC13   AC14   200m   NA
|Differential signal data for cell ACSPCIE_RX
|LJCB_CLKP   LJCB_CLKN
AE13   AF14   150m   NA   NA   NA
|Differential signal data for cell HDMITXPHY
|HDMI1_CLOCKX   HDMI1_CLOCKY
AG14   AH15   0.0V   0.0s
|HDMI1_DATA0X   HDMI1_DATA0Y
AG15   AH16   0.0V   0.0s
|HDMI1_DATA2X   HDMI1_DATA2Y
AG18   AH19   0.0V   0.0s
|HDMI1_DATA1X   HDMI1_DATA1Y
AG17   AH18   0.0V   0.0s
|Differential signal data for cell GANGARX
|SATA1_RXP0   SATA1_RXN0
AG5   AH6   100mV  NA
|PCIE_RXP0   PCIE_RXN0
AH12   AG11   100mV  NA
|PCIE_RXP1   PCIE_RXN1
AH9   AG8   100mV  NA
|USB_RXP0   USB_RXN0
AH4   AG3   100mV  NA
|   Usage OUTPUT#1.35/1.5/1.8###DDR_DIFFIOPB_V.PADN
|   Base model DDR_DIFFIOPB_V
[Model Selector] Selector_1
SR011_DRV48_1P8_M#242 I/O,1.8V,SR011_DRV48_1P8
SR010_DRV48_1P8_M#243 I/O,1.8V,SR010_DRV48_1P8
SR101_DRV48_1P8_M#244 I/O,1.8V,SR101_DRV48_1P8
SR100_DRV48_1P8_M#245 I/O,1.8V,SR100_DRV48_1P8
SR110_DRV48_1P8_M#246 I/O,1.8V,SR110_DRV48_1P8
SR111_DRV48_1P8_M#247 I/O,1.8V,SR111_DRV48_1P8
SR001_DRV48_1P8_M#248 I/O,1.8V,SR001_DRV48_1P8
SR000_DRV48_1P8_M#249 I/O,1.8V,SR000_DRV48_1P8
SR011_DRV40_1P8_M#250 I/O,1.8V,SR011_DRV40_1P8
SR010_DRV40_1P8_M#251 I/O,1.8V,SR010_DRV40_1P8
SR101_DRV40_1P8_M#252 I/O,1.8V,SR101_DRV40_1P8
SR100_DRV40_1P8_M#253 I/O,1.8V,SR100_DRV40_1P8
SR110_DRV40_1P8_M#254 I/O,1.8V,SR110_DRV40_1P8
SR111_DRV40_1P8_M#255 I/O,1.8V,SR111_DRV40_1P8
SR001_DRV40_1P8_M#256 I/O,1.8V,SR001_DRV40_1P8
SR000_DRV40_1P8_M#257 I/O,1.8V,SR000_DRV40_1P8
SR011_DRV34_1P8_M#258 I/O,1.8V,SR011_DRV34_1P8
SR010_DRV34_1P8_M#259 I/O,1.8V,SR010_DRV34_1P8
SR101_DRV34_1P8_M#260 I/O,1.8V,SR101_DRV34_1P8
SR100_DRV34_1P8_M#261 I/O,1.8V,SR100_DRV34_1P8
SR110_DRV34_1P8_M#262 I/O,1.8V,SR110_DRV34_1P8
SR111_DRV34_1P8_M#263 I/O,1.8V,SR111_DRV34_1P8
SR001_DRV34_1P8_M#264 I/O,1.8V,SR001_DRV34_1P8
SR000_DRV34_1P8_M#265 I/O,1.8V,SR000_DRV34_1P8
SR011_DRV40_1P5_M#275 I/O,1.5V,SR011_DRV40_1P5
SR010_DRV40_1P5_M#276 I/O,1.5V,SR010_DRV40_1P5
SR101_DRV40_1P5_M#277 I/O,1.5V,SR101_DRV40_1P5
SR100_DRV40_1P5_M#278 I/O,1.5V,SR100_DRV40_1P5
SR110_DRV40_1P5_M#279 I/O,1.5V,SR110_DRV40_1P5
SR111_DRV40_1P5_M#280 I/O,1.5V,SR111_DRV40_1P5
SR001_DRV40_1P5_M#281 I/O,1.5V,SR001_DRV40_1P5
SR000_DRV40_1P5_M#282 I/O,1.5V,SR000_DRV40_1P5
SR011_DRV34_1P5_M#283 I/O,1.5V,SR011_DRV34_1P5
SR010_DRV34_1P5_M#284 I/O,1.5V,SR010_DRV34_1P5
SR101_DRV34_1P5_M#285 I/O,1.5V,SR101_DRV34_1P5
SR100_DRV34_1P5_M#286 I/O,1.5V,SR100_DRV34_1P5
SR110_DRV34_1P5_M#287 I/O,1.5V,SR110_DRV34_1P5
SR111_DRV34_1P5_M#288 I/O,1.5V,SR111_DRV34_1P5
SR001_DRV34_1P5_M#289 I/O,1.5V,SR001_DRV34_1P5
SR000_DRV34_1P5_M#290 I/O,1.5V,SR000_DRV34_1P5
SR011_DRV48_1P5_M#291 I/O,1.5V,SR011_DRV48_1P5
SR010_DRV48_1P5_M#292 I/O,1.5V,SR010_DRV48_1P5
SR101_DRV48_1P5_M#293 I/O,1.5V,SR101_DRV48_1P5
SR100_DRV48_1P5_M#294 I/O,1.5V,SR100_DRV48_1P5
SR110_DRV48_1P5_M#295 I/O,1.5V,SR110_DRV48_1P5
SR111_DRV48_1P5_M#296 I/O,1.5V,SR111_DRV48_1P5
SR001_DRV48_1P5_M#297 I/O,1.5V,SR001_DRV48_1P5
SR000_DRV48_1P5_M#298 I/O,1.5V,SR000_DRV48_1P5
SR011_DRV40_1P35_M#299 I/O,1.35V,SR011_DRV40_1P35
SR010_DRV40_1P35_M#300 I/O,1.35V,SR010_DRV40_1P35
SR101_DRV40_1P35_M#301 I/O,1.35V,SR101_DRV40_1P35
SR100_DRV40_1P35_M#302 I/O,1.35V,SR100_DRV40_1P35
SR110_DRV40_1P35_M#303 I/O,1.35V,SR110_DRV40_1P35
SR111_DRV40_1P35_M#304 I/O,1.35V,SR111_DRV40_1P35
SR001_DRV40_1P35_M#305 I/O,1.35V,SR001_DRV40_1P35
SR000_DRV40_1P35_M#306 I/O,1.35V,SR000_DRV40_1P35
SR011_DRV34_1P35_M#307 I/O,1.35V,SR011_DRV34_1P35
SR010_DRV34_1P35_M#308 I/O,1.35V,SR010_DRV34_1P35
SR101_DRV34_1P35_M#309 I/O,1.35V,SR101_DRV34_1P35
SR100_DRV34_1P35_M#310 I/O,1.35V,SR100_DRV34_1P35
SR110_DRV34_1P35_M#311 I/O,1.35V,SR110_DRV34_1P35
SR111_DRV34_1P35_M#312 I/O,1.35V,SR111_DRV34_1P35
SR001_DRV34_1P35_M#313 I/O,1.35V,SR001_DRV34_1P35
SR000_DRV34_1P35_M#314 I/O,1.35V,SR000_DRV34_1P35
SR011_DRV48_1P35_M#315 I/O,1.35V,SR011_DRV48_1P35
SR010_DRV48_1P35_M#316 I/O,1.35V,SR010_DRV48_1P35
SR101_DRV48_1P35_M#317 I/O,1.35V,SR101_DRV48_1P35
SR100_DRV48_1P35_M#318 I/O,1.35V,SR100_DRV48_1P35
SR110_DRV48_1P35_M#319 I/O,1.35V,SR110_DRV48_1P35
SR111_DRV48_1P35_M#320 I/O,1.35V,SR111_DRV48_1P35
SR001_DRV48_1P35_M#321 I/O,1.35V,SR001_DRV48_1P35
SR000_DRV48_1P35_M#322 I/O,1.35V,SR000_DRV48_1P35
|   Usage INPUT#1.8###BMLBLVDS18_SSCEH.PAD
|   Base model BMLBLVDS18_SSCEH
[Model Selector] Selector_2
LVDS_RX_MODE_5P_1P8_M#696 INPUT,1.8V,LVDS MODE,IND,5%,LVDS_RX_MODE_5P_1P8
LVDS_RX_MODE_10P_1P8_M#697 INPUT,1.8V,LVDS MODE,IND,10%,LVDS_RX_MODE_10P_1P8
|   Usage OUTPUT#1.8/3.3###BC1833DV40DCPBFBP1811_SSCEV.PAD
|   Base model BC1833DV40DCPBFBP1811_SSCEV
[Model Selector] Selector_3
BC40D_V_10P_!SC1_1P8_M#527 I/O,1.8V,40D CLASS MODE FAST MODE,IND,10 PERCENT%,BC40D_V_10P_!SC1_1P8
BC40D_V_10P_SC1_1P8_M#528 I/O,1.8V,40C CLASS MODE SLOW MODE,IND,10 PERCENT%,BC40D_V_10P_SC1_1P8
BC40D_V_5P_!SC1_1P8_M#529 I/O,1.8V,40D CLASS MODE FAST MODE,IND,5 PERCENT%,BC40D_V_5P_!SC1_1P8
BC40D_V_5P_SC1_1P8_M#530 I/O,1.8V,40C CLASS MODE SLOW MODE,IND,5 PERCENT%,BC40D_V_5P_SC1_1P8
BC40D_V_10P_!SC1_3P3_M#531 I/O,3.3V,40D CLASS MODE FAST MODE,IND,10 PERCENT%,BC40D_V_10P_!SC1_3P3
BC40D_V_10P_SC1_3P3_M#532 I/O,3.3V,40C CLASS MODE SLOW MODE,IND,10 PERCENT%,BC40D_V_10P_SC1_3P3
BC40D_V_5P_!SC1_3P3_M#533 I/O,3.3V,40D CLASS MODE FAST MODE,IND,5 PERCENT%,BC40D_V_5P_!SC1_3P3
BC40D_V_5P_SC1_3P3_M#534 I/O,3.3V,40C CLASS MODE SLOW MODE,IND,5 PERCENT%,BC40D_V_5P_SC1_3P3
|   Usage I/O#1.8/3.3###BC1833DV40DCPBFBP1811_SSCEH.PAD
|   Base model BC1833DV40DCPBFBP1811_SSCEH
[Model Selector] Selector_4
BC40D_H_10P_!SC1_1P8_M#327 I/O,1.8V,40D CLASS MODE FAST MODE,IND,10 PERCENT%,BC40D_H_10P_!SC1_1P8
BC40D_H_10P_SC1_1P8_M#328 I/O,1.8V,40C CLASS MODE SLOW MODE,IND,10 PERCENT%,BC40D_H_10P_SC1_1P8
BC40D_H_5P_!SC1_1P8_M#329 I/O,1.8V,40D CLASS MODE FAST MODE,IND,5 PERCENT%,BC40D_H_5P_!SC1_1P8
BC40D_H_5P_SC1_1P8_M#330 I/O,1.8V,40C CLASS MODE SLOW MODE,IND,5 PERCENT%,BC40D_H_5P_SC1_1P8
BC40D_H_10P_!SC1_3P3_M#331 I/O,3.3V,40D CLASS MODE FAST MODE,IND,10 PERCENT%,BC40D_H_10P_!SC1_3P3
BC40D_H_10P_SC1_3P3_M#332 I/O,3.3V,40C CLASS MODE SLOW MODE,IND,10 PERCENT%,BC40D_H_10P_SC1_3P3
BC40D_H_5P_!SC1_3P3_M#333 I/O,3.3V,40D CLASS MODE FAST MODE,IND,5 PERCENT%,BC40D_H_5P_!SC1_3P3
BC40D_H_5P_SC1_3P3_M#334 I/O,3.3V,40C CLASS MODE SLOW MODE,IND,5 PERCENT%,BC40D_H_5P_SC1_3P3
|   Usage I/O#1.8/3###SDIO1833PB_H.PAD
|   Base model SDIO1833PB_H
[Model Selector] Selector_5
50OHMS_3_M#507 I/O,3V,50OHMS_3
66OHMS_3_M#508 I/O,3V,66OHMS_3
33OHMS_3_M#509 I/O,3V,33OHMS_3
100OHMS_3_M#510 I/O,3V,100OHMS_3
50OHMS_1P8_M#511 I/O,1.8V,50OHMS_1P8
66OHMS_1P8_M#512 I/O,1.8V,66OHMS_1P8
33OHMS_1P8_M#513 I/O,1.8V,33OHMS_1P8
100OHMS_1P8_M#514 I/O,1.8V,100OHMS_1P8
|   Usage OUTPUT#1.35/1.5/1.8###DDR_DIFFIOPB_V.PADP
|   Base model DDR_DIFFIOPB_V
[Model Selector] Selector_6
SR011_DRV48_1P8_M#242 I/O,1.8V,SR011_DRV48_1P8
SR010_DRV48_1P8_M#243 I/O,1.8V,SR010_DRV48_1P8
SR101_DRV48_1P8_M#244 I/O,1.8V,SR101_DRV48_1P8
SR100_DRV48_1P8_M#245 I/O,1.8V,SR100_DRV48_1P8
SR110_DRV48_1P8_M#246 I/O,1.8V,SR110_DRV48_1P8
SR111_DRV48_1P8_M#247 I/O,1.8V,SR111_DRV48_1P8
SR001_DRV48_1P8_M#248 I/O,1.8V,SR001_DRV48_1P8
SR000_DRV48_1P8_M#249 I/O,1.8V,SR000_DRV48_1P8
SR011_DRV40_1P8_M#250 I/O,1.8V,SR011_DRV40_1P8
SR010_DRV40_1P8_M#251 I/O,1.8V,SR010_DRV40_1P8
SR101_DRV40_1P8_M#252 I/O,1.8V,SR101_DRV40_1P8
SR100_DRV40_1P8_M#253 I/O,1.8V,SR100_DRV40_1P8
SR110_DRV40_1P8_M#254 I/O,1.8V,SR110_DRV40_1P8
SR111_DRV40_1P8_M#255 I/O,1.8V,SR111_DRV40_1P8
SR001_DRV40_1P8_M#256 I/O,1.8V,SR001_DRV40_1P8
SR000_DRV40_1P8_M#257 I/O,1.8V,SR000_DRV40_1P8
SR011_DRV34_1P8_M#258 I/O,1.8V,SR011_DRV34_1P8
SR010_DRV34_1P8_M#259 I/O,1.8V,SR010_DRV34_1P8
SR101_DRV34_1P8_M#260 I/O,1.8V,SR101_DRV34_1P8
SR100_DRV34_1P8_M#261 I/O,1.8V,SR100_DRV34_1P8
SR110_DRV34_1P8_M#262 I/O,1.8V,SR110_DRV34_1P8
SR111_DRV34_1P8_M#263 I/O,1.8V,SR111_DRV34_1P8
SR001_DRV34_1P8_M#264 I/O,1.8V,SR001_DRV34_1P8
SR000_DRV34_1P8_M#265 I/O,1.8V,SR000_DRV34_1P8
SR011_DRV40_1P5_M#275 I/O,1.5V,SR011_DRV40_1P5
SR010_DRV40_1P5_M#276 I/O,1.5V,SR010_DRV40_1P5
SR101_DRV40_1P5_M#277 I/O,1.5V,SR101_DRV40_1P5
SR100_DRV40_1P5_M#278 I/O,1.5V,SR100_DRV40_1P5
SR110_DRV40_1P5_M#279 I/O,1.5V,SR110_DRV40_1P5
SR111_DRV40_1P5_M#280 I/O,1.5V,SR111_DRV40_1P5
SR001_DRV40_1P5_M#281 I/O,1.5V,SR001_DRV40_1P5
SR000_DRV40_1P5_M#282 I/O,1.5V,SR000_DRV40_1P5
SR011_DRV34_1P5_M#283 I/O,1.5V,SR011_DRV34_1P5
SR010_DRV34_1P5_M#284 I/O,1.5V,SR010_DRV34_1P5
SR101_DRV34_1P5_M#285 I/O,1.5V,SR101_DRV34_1P5
SR100_DRV34_1P5_M#286 I/O,1.5V,SR100_DRV34_1P5
SR110_DRV34_1P5_M#287 I/O,1.5V,SR110_DRV34_1P5
SR111_DRV34_1P5_M#288 I/O,1.5V,SR111_DRV34_1P5
SR001_DRV34_1P5_M#289 I/O,1.5V,SR001_DRV34_1P5
SR000_DRV34_1P5_M#290 I/O,1.5V,SR000_DRV34_1P5
SR011_DRV48_1P5_M#291 I/O,1.5V,SR011_DRV48_1P5
SR010_DRV48_1P5_M#292 I/O,1.5V,SR010_DRV48_1P5
SR101_DRV48_1P5_M#293 I/O,1.5V,SR101_DRV48_1P5
SR100_DRV48_1P5_M#294 I/O,1.5V,SR100_DRV48_1P5
SR110_DRV48_1P5_M#295 I/O,1.5V,SR110_DRV48_1P5
SR111_DRV48_1P5_M#296 I/O,1.5V,SR111_DRV48_1P5
SR001_DRV48_1P5_M#297 I/O,1.5V,SR001_DRV48_1P5
SR000_DRV48_1P5_M#298 I/O,1.5V,SR000_DRV48_1P5
SR011_DRV40_1P35_M#299 I/O,1.35V,SR011_DRV40_1P35
SR010_DRV40_1P35_M#300 I/O,1.35V,SR010_DRV40_1P35
SR101_DRV40_1P35_M#301 I/O,1.35V,SR101_DRV40_1P35
SR100_DRV40_1P35_M#302 I/O,1.35V,SR100_DRV40_1P35
SR110_DRV40_1P35_M#303 I/O,1.35V,SR110_DRV40_1P35
SR111_DRV40_1P35_M#304 I/O,1.35V,SR111_DRV40_1P35
SR001_DRV40_1P35_M#305 I/O,1.35V,SR001_DRV40_1P35
SR000_DRV40_1P35_M#306 I/O,1.35V,SR000_DRV40_1P35
SR011_DRV34_1P35_M#307 I/O,1.35V,SR011_DRV34_1P35
SR010_DRV34_1P35_M#308 I/O,1.35V,SR010_DRV34_1P35
SR101_DRV34_1P35_M#309 I/O,1.35V,SR101_DRV34_1P35
SR100_DRV34_1P35_M#310 I/O,1.35V,SR100_DRV34_1P35
SR110_DRV34_1P35_M#311 I/O,1.35V,SR110_DRV34_1P35
SR111_DRV34_1P35_M#312 I/O,1.35V,SR111_DRV34_1P35
SR001_DRV34_1P35_M#313 I/O,1.35V,SR001_DRV34_1P35
SR000_DRV34_1P35_M#314 I/O,1.35V,SR000_DRV34_1P35
SR011_DRV48_1P35_M#315 I/O,1.35V,SR011_DRV48_1P35
SR010_DRV48_1P35_M#316 I/O,1.35V,SR010_DRV48_1P35
SR101_DRV48_1P35_M#317 I/O,1.35V,SR101_DRV48_1P35
SR100_DRV48_1P35_M#318 I/O,1.35V,SR100_DRV48_1P35
SR110_DRV48_1P35_M#319 I/O,1.35V,SR110_DRV48_1P35
SR111_DRV48_1P35_M#320 I/O,1.35V,SR111_DRV48_1P35
SR001_DRV48_1P35_M#321 I/O,1.35V,SR001_DRV48_1P35
SR000_DRV48_1P35_M#322 I/O,1.35V,SR000_DRV48_1P35
|   Usage OUTPUT#X###USB3_PCIEGEN1_PCIEGEN2_TX.TXN
|   Base model USB3_PCIEGEN1_PCIEGEN2_TX
[Model Selector] Selector_7
USB3_TX_FS_NO_DEEMPHASIS_M#720 3-STATE,1.1V,USB3_TX_FS_NO_DEEMPHASIS
USB3_TX_FS_3p5_DEEMPHASIS_M#721 3-STATE,1.1V,USB3_TX_FS_3p5_DEEMPHASIS
USB3_TX_HS_NO_DEEMPHASIS_M#722 3-STATE,1.1V,USB3_TX_HS_NO_DEEMPHASIS
PCIEGEN1_TX_FS_NO_DEEMPHASIS_1p2v_M#723 3-STATE,1.1V,PCIEGEN1_TX_FS_NO_DEEMPHASIS_1p2v
PCIEGEN1_TX_FS_NO_DEEMPHASIS_0p8v_M#724 3-STATE,1.1V,PCIEGEN1_TX_FS_NO_DEEMPHASIS_0p8v
PCIEGEN1_TX_FS_NO_DEEMPHASIS_0p6v_M#725 3-STATE,1.1V,PCIEGEN1_TX_FS_NO_DEEMPHASIS_0p6v
PCIEGEN1_TX_FS_NO_DEEMPHASIS_0p4v_M#726 3-STATE,1.1V,PCIEGEN1_TX_FS_NO_DEEMPHASIS_0p4v
PCIEGEN1_TX_FS_3p5_DEEMPHASIS_1p2v_M#727 3-STATE,1.1V,PCIEGEN1_TX_FS_3p5_DEEMPHASIS_1p2v
PCIEGEN1_TX_FS_3p5_DEEMPHASIS_0p8v_M#728 3-STATE,1.1V,PCIEGEN1_TX_FS_3p5_DEEMPHASIS_0p8v
PCIEGEN1_TX_FS_3p5_DEEMPHASIS_0p6v_M#729 3-STATE,1.1V,PCIEGEN1_TX_FS_3p5_DEEMPHASIS_0p6v
PCIEGEN1_TX_FS_3p5_DEEMPHASIS_0p4v_M#730 3-STATE,1.1V,PCIEGEN1_TX_FS_3p5_DEEMPHASIS_0p4v
PCIEGEN1_TX_HS_NO_DEEMPHASIS_0p6v_M#731 3-STATE,1.1V,PCIEGEN1_TX_HS_NO_DEEMPHASIS_0p6v
PCIEGEN1_TX_HS_NO_DEEMPHASIS_0p4v_M#732 3-STATE,1.1V,PCIEGEN1_TX_HS_NO_DEEMPHASIS_0p4v
PCIEGEN1_TX_HS_NO_DEEMPHASIS_0p3v_M#733 3-STATE,1.1V,PCIEGEN1_TX_HS_NO_DEEMPHASIS_0p3v
PCIEGEN1_TX_HS_NO_DEEMPHASIS_0p2v_M#734 3-STATE,1.1V,PCIEGEN1_TX_HS_NO_DEEMPHASIS_0p2v
PCIEGEN2_TX_FS_NO_DEEMPHASIS_1p2v_M#735 3-STATE,1.1V,PCIEGEN2_TX_FS_NO_DEEMPHASIS_1p2v
PCIEGEN2_TX_FS_NO_DEEMPHASIS_0p8v_M#736 3-STATE,1.1V,PCIEGEN2_TX_FS_NO_DEEMPHASIS_0p8v
PCIEGEN2_TX_FS_NO_DEEMPHASIS_0p6v_M#737 3-STATE,1.1V,PCIEGEN2_TX_FS_NO_DEEMPHASIS_0p6v
PCIEGEN2_TX_FS_NO_DEEMPHASIS_0p4v_M#738 3-STATE,1.1V,PCIEGEN2_TX_FS_NO_DEEMPHASIS_0p4v
PCIEGEN2_TX_FS_3p5_DEEMPHASIS_1p2v_M#739 3-STATE,1.1V,PCIEGEN2_TX_FS_3p5_DEEMPHASIS_1p2v
PCIEGEN2_TX_FS_3p5_DEEMPHASIS_0p8v_M#740 3-STATE,1.1V,PCIEGEN2_TX_FS_3p5_DEEMPHASIS_0p8v
PCIEGEN2_TX_FS_3p5_DEEMPHASIS_0p6v_M#741 3-STATE,1.1V,PCIEGEN2_TX_FS_3p5_DEEMPHASIS_0p6v
PCIEGEN2_TX_FS_3p5_DEEMPHASIS_0p4v_M#742 3-STATE,1.1V,PCIEGEN2_TX_FS_3p5_DEEMPHASIS_0p4v
PCIEGEN2_TX_FS_6p0_DEEMPHASIS_1p2v_M#743 3-STATE,1.1V,PCIEGEN2_TX_FS_6p0_DEEMPHASIS_1p2v
PCIEGEN2_TX_FS_6p0_DEEMPHASIS_0p8v_M#744 3-STATE,1.1V,PCIEGEN2_TX_FS_6p0_DEEMPHASIS_0p8v
PCIEGEN2_TX_FS_6p0_DEEMPHASIS_0p6v_M#745 3-STATE,1.1V,PCIEGEN2_TX_FS_6p0_DEEMPHASIS_0p6v
PCIEGEN2_TX_FS_6p0_DEEMPHASIS_0p4v_M#746 3-STATE,1.1V,PCIEGEN2_TX_FS_6p0_DEEMPHASIS_0p4v
PCIEGEN2_TX_HS_NO_DEEMPHASIS_0p6v_M#747 3-STATE,1.1V,PCIEGEN2_TX_HS_NO_DEEMPHASIS_0p6v
PCIEGEN2_TX_HS_NO_DEEMPHASIS_0p4v_M#748 3-STATE,1.1V,PCIEGEN2_TX_HS_NO_DEEMPHASIS_0p4v
PCIEGEN2_TX_HS_NO_DEEMPHASIS_0p3v_M#749 3-STATE,1.1V,PCIEGEN2_TX_HS_NO_DEEMPHASIS_0p3v
PCIEGEN2_TX_HS_NO_DEEMPHASIS_0p2v_M#750 3-STATE,1.1V,PCIEGEN2_TX_HS_NO_DEEMPHASIS_0p2v
|   Usage INPUT#1.8/3.3###BC1833DV40DCPBFBP1811_SSCEV.PAD
|   Base model BC1833DV40DCPBFBP1811_SSCEV
[Model Selector] Selector_8
BC40D_V_10P_!SC1_1P8_M#527 I/O,1.8V,40D CLASS MODE FAST MODE,IND,10 PERCENT%,BC40D_V_10P_!SC1_1P8
BC40D_V_10P_SC1_1P8_M#528 I/O,1.8V,40C CLASS MODE SLOW MODE,IND,10 PERCENT%,BC40D_V_10P_SC1_1P8
BC40D_V_5P_!SC1_1P8_M#529 I/O,1.8V,40D CLASS MODE FAST MODE,IND,5 PERCENT%,BC40D_V_5P_!SC1_1P8
BC40D_V_5P_SC1_1P8_M#530 I/O,1.8V,40C CLASS MODE SLOW MODE,IND,5 PERCENT%,BC40D_V_5P_SC1_1P8
BC40D_V_10P_!SC1_3P3_M#531 I/O,3.3V,40D CLASS MODE FAST MODE,IND,10 PERCENT%,BC40D_V_10P_!SC1_3P3
BC40D_V_10P_SC1_3P3_M#532 I/O,3.3V,40C CLASS MODE SLOW MODE,IND,10 PERCENT%,BC40D_V_10P_SC1_3P3
BC40D_V_5P_!SC1_3P3_M#533 I/O,3.3V,40D CLASS MODE FAST MODE,IND,5 PERCENT%,BC40D_V_5P_!SC1_3P3
BC40D_V_5P_SC1_3P3_M#534 I/O,3.3V,40C CLASS MODE SLOW MODE,IND,5 PERCENT%,BC40D_V_5P_SC1_3P3
|   Usage I/O#1.8###BMLBLVDS18_SSCEH.PAD
|   Base model BMLBLVDS18_SSCEH
[Model Selector] Selector_9
LVDS_RX_MODE_5P_1P8_M#696 INPUT,1.8V,LVDS MODE,IND,5%,LVDS_RX_MODE_5P_1P8
LVDS_RX_MODE_10P_1P8_M#697 INPUT,1.8V,LVDS MODE,IND,10%,LVDS_RX_MODE_10P_1P8
LVDS_TXMODE_5P_1P8_M#698 3-STATE,1.8V,8MA,IND,5%,LVDS_TXMODE_5P_1P8
LVDS_TXMODE_10P_1P8_M#699 3-STATE,1.8V,8MA,IND,10%,LVDS_TXMODE_10P_1P8
|   Usage I/O#X###USB2PHYCORE_HMAV10GS80.DP
|   Base model USB2PHYCORE_HMAV10GS80
[Model Selector] Selector_10
fsdp_tx_M#700 3-STATE,3.3000V,fsdp_tx
lsdp_50pf_tx_M#702 3-STATE,3.3000V,lsdp_50pf_tx
lsdp_200pf_tx_M#704 3-STATE,3.3000V,lsdp_200pf_tx
lsdp_400pf_tx_M#706 3-STATE,3.3000V,lsdp_400pf_tx
lsdp_600pf_tx_M#708 3-STATE,3.3000V,lsdp_600pf_tx
fsrx_M#710 INPUT,3.3V,fsrx
hsdp_tx_M#711 3-STATE,0.8000V,hsdp_tx
hsrx_M#713 INPUT,3.3V,hsrx
|   Usage OUTPUT#1.35/1.5/1.8###DDR_SEIOPB_H.PAD
|   Base model DDR_SEIOPB_H
[Model Selector] Selector_11
SR011_DRV48_1P8_M#426 I/O,1.8V,SR011_DRV48_1P8
SR010_DRV48_1P8_M#427 I/O,1.8V,SR010_DRV48_1P8
SR101_DRV48_1P8_M#428 I/O,1.8V,SR101_DRV48_1P8
SR100_DRV48_1P8_M#429 I/O,1.8V,SR100_DRV48_1P8
SR110_DRV48_1P8_M#430 I/O,1.8V,SR110_DRV48_1P8
SR111_DRV48_1P8_M#431 I/O,1.8V,SR111_DRV48_1P8
SR001_DRV48_1P8_M#432 I/O,1.8V,SR001_DRV48_1P8
SR000_DRV48_1P8_M#433 I/O,1.8V,SR000_DRV48_1P8
SR011_DRV40_1P8_M#434 I/O,1.8V,SR011_DRV40_1P8
SR010_DRV40_1P8_M#435 I/O,1.8V,SR010_DRV40_1P8
SR101_DRV40_1P8_M#436 I/O,1.8V,SR101_DRV40_1P8
SR100_DRV40_1P8_M#437 I/O,1.8V,SR100_DRV40_1P8
SR110_DRV40_1P8_M#438 I/O,1.8V,SR110_DRV40_1P8
SR111_DRV40_1P8_M#439 I/O,1.8V,SR111_DRV40_1P8
SR001_DRV40_1P8_M#440 I/O,1.8V,SR001_DRV40_1P8
SR000_DRV40_1P8_M#441 I/O,1.8V,SR000_DRV40_1P8
SR011_DRV34_1P8_M#442 I/O,1.8V,SR011_DRV34_1P8
SR010_DRV34_1P8_M#443 I/O,1.8V,SR010_DRV34_1P8
SR101_DRV34_1P8_M#444 I/O,1.8V,SR101_DRV34_1P8
SR100_DRV34_1P8_M#445 I/O,1.8V,SR100_DRV34_1P8
SR110_DRV34_1P8_M#446 I/O,1.8V,SR110_DRV34_1P8
SR111_DRV34_1P8_M#447 I/O,1.8V,SR111_DRV34_1P8
SR001_DRV34_1P8_M#448 I/O,1.8V,SR001_DRV34_1P8
SR000_DRV34_1P8_M#449 I/O,1.8V,SR000_DRV34_1P8
SR011_DRV40_1P5_M#459 I/O,1.5V,SR011_DRV40_1P5
SR010_DRV40_1P5_M#460 I/O,1.5V,SR010_DRV40_1P5
SR101_DRV40_1P5_M#461 I/O,1.5V,SR101_DRV40_1P5
SR100_DRV40_1P5_M#462 I/O,1.5V,SR100_DRV40_1P5
SR110_DRV40_1P5_M#463 I/O,1.5V,SR110_DRV40_1P5
SR111_DRV40_1P5_M#464 I/O,1.5V,SR111_DRV40_1P5
SR001_DRV40_1P5_M#465 I/O,1.5V,SR001_DRV40_1P5
SR000_DRV40_1P5_M#466 I/O,1.5V,SR000_DRV40_1P5
SR011_DRV34_1P5_M#467 I/O,1.5V,SR011_DRV34_1P5
SR010_DRV34_1P5_M#468 I/O,1.5V,SR010_DRV34_1P5
SR101_DRV34_1P5_M#469 I/O,1.5V,SR101_DRV34_1P5
SR100_DRV34_1P5_M#470 I/O,1.5V,SR100_DRV34_1P5
SR110_DRV34_1P5_M#471 I/O,1.5V,SR110_DRV34_1P5
SR111_DRV34_1P5_M#472 I/O,1.5V,SR111_DRV34_1P5
SR001_DRV34_1P5_M#473 I/O,1.5V,SR001_DRV34_1P5
SR000_DRV34_1P5_M#474 I/O,1.5V,SR000_DRV34_1P5
SR011_DRV48_1P5_M#475 I/O,1.5V,SR011_DRV48_1P5
SR010_DRV48_1P5_M#476 I/O,1.5V,SR010_DRV48_1P5
SR101_DRV48_1P5_M#477 I/O,1.5V,SR101_DRV48_1P5
SR100_DRV48_1P5_M#478 I/O,1.5V,SR100_DRV48_1P5
SR110_DRV48_1P5_M#479 I/O,1.5V,SR110_DRV48_1P5
SR111_DRV48_1P5_M#480 I/O,1.5V,SR111_DRV48_1P5
SR001_DRV48_1P5_M#481 I/O,1.5V,SR001_DRV48_1P5
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| Models and submodels in the file (415): SR011_DRV48_1P8_M#81 (I/O), SR010_DRV48_1P8_M#82 (I/O), SR101_DRV48_1P8_M#83 (I/O), SR100_DRV48_1P8_M#84 (I/O), SR110_DRV48_1P8_M#85 (I/O), SR111_DRV48_1P8_M#86 (I/O), SR001_DRV48_1P8_M#87 (I/O), SR000_DRV48_1P8_M#88 (I/O), SR011_DRV40_1P8_M#89 (I/O), SR010_DRV40_1P8_M#90 (I/O), SR101_DRV40_1P8_M#91 (I/O), SR100_DRV40_1P8_M#92 (I/O), SR110_DRV40_1P8_M#93 (I/O), SR111_DRV40_1P8_M#94 (I/O), SR001_DRV40_1P8_M#95 (I/O), SR000_DRV40_1P8_M#96 (I/O), SR011_DRV34_1P8_M#97 (I/O), SR010_DRV34_1P8_M#98 (I/O), SR101_DRV34_1P8_M#99 (I/O), SR100_DRV34_1P8_M#100 (I/O), SR110_DRV34_1P8_M#101 (I/O), SR111_DRV34_1P8_M#102 (I/O), SR001_DRV34_1P8_M#103 (I/O), SR000_DRV34_1P8_M#104 (I/O), SR011_DRV40_1P5_M#114 (I/O), SR010_DRV40_1P5_M#115 (I/O), SR101_DRV40_1P5_M#116 (I/O), SR100_DRV40_1P5_M#117 (I/O), SR110_DRV40_1P5_M#118 (I/O), SR111_DRV40_1P5_M#119 (I/O), SR001_DRV40_1P5_M#120 (I/O), SR000_DRV40_1P5_M#121 (I/O), SR011_DRV34_1P5_M#122 (I/O), SR010_DRV34_1P5_M#123 (I/O), SR101_DRV34_1P5_M#124 (I/O), SR100_DRV34_1P5_M#125 (I/O), SR110_DRV34_1P5_M#126 (I/O), SR111_DRV34_1P5_M#127 (I/O), SR001_DRV34_1P5_M#128 (I/O), SR000_DRV34_1P5_M#129 (I/O), SR011_DRV48_1P5_M#130 (I/O), SR010_DRV48_1P5_M#131 (I/O), SR101_DRV48_1P5_M#132 (I/O), SR100_DRV48_1P5_M#133 (I/O), SR110_DRV48_1P5_M#134 (I/O), SR111_DRV48_1P5_M#135 (I/O), SR001_DRV48_1P5_M#136 (I/O), SR000_DRV48_1P5_M#137 (I/O), SR011_DRV40_1P35_M#138 (I/O), SR010_DRV40_1P35_M#139 (I/O), SR101_DRV40_1P35_M#140 (I/O), SR100_DRV40_1P35_M#141 (I/O), SR110_DRV40_1P35_M#142 (I/O), SR111_DRV40_1P35_M#143 (I/O), SR001_DRV40_1P35_M#144 (I/O), SR000_DRV40_1P35_M#145 (I/O), SR011_DRV34_1P35_M#146 (I/O), SR010_DRV34_1P35_M#147 (I/O), SR101_DRV34_1P35_M#148 (I/O), SR100_DRV34_1P35_M#149 (I/O), SR110_DRV34_1P35_M#150 (I/O), SR111_DRV34_1P35_M#151 (I/O), SR001_DRV34_1P35_M#152 (I/O), SR000_DRV34_1P35_M#153 (I/O), SR011_DRV48_1P35_M#154 (I/O), SR010_DRV48_1P35_M#155 (I/O), SR101_DRV48_1P35_M#156 (I/O), SR100_DRV48_1P35_M#157 (I/O), SR110_DRV48_1P35_M#158 (I/O), SR111_DRV48_1P35_M#159 (I/O), SR001_DRV48_1P35_M#160 (I/O), SR000_DRV48_1P35_M#161 (I/O), SR011_DRV48_1P8_M#242 (I/O), SR010_DRV48_1P8_M#243 (I/O), SR101_DRV48_1P8_M#244 (I/O), SR100_DRV48_1P8_M#245 (I/O), SR110_DRV48_1P8_M#246 (I/O), SR111_DRV48_1P8_M#247 (I/O), SR001_DRV48_1P8_M#248 (I/O), SR000_DRV48_1P8_M#249 (I/O)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
